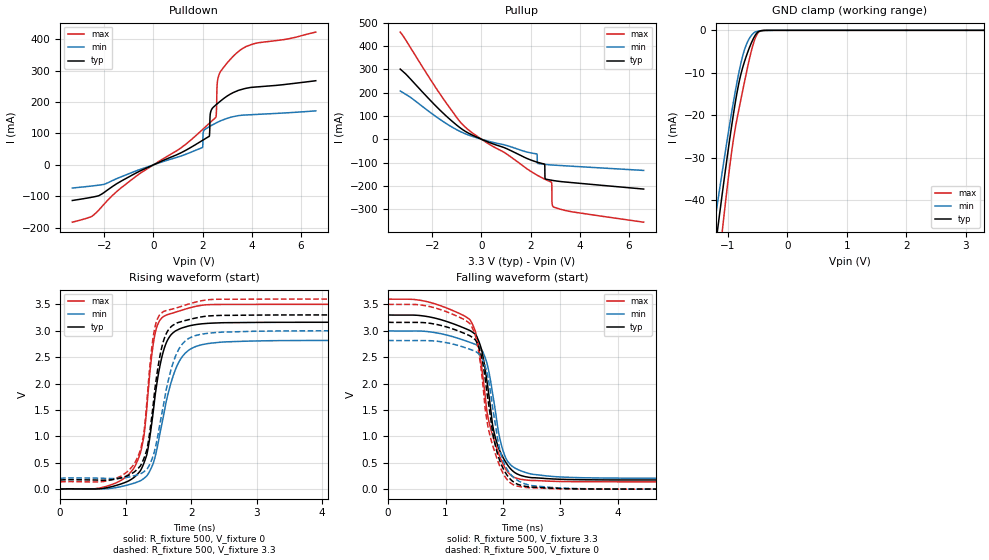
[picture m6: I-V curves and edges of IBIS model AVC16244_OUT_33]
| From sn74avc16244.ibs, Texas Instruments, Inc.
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[Model]   AVC16244_OUT_33
Model_type  3-state
Enable   Active-Low
Vref =   0
Rref =   500
Cref =   50p
Vmeas =   1.5
| variable   typ   min   max
C_comp   4.23pF   3.26pF   5.24pF
| C_pullup   8.74pF   0.03pF   34.91pF
| C_pulldown   15.41pF   1.21pF   46.75pF
| C_tri-state   4.23pF   3.26pF   5.24pF
[Temperature Range]   40   100   -40
| Ambient temperature   25   85   -40
[Voltage range]   3.3   3   3.6
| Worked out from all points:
|   slope of the pulldown table from 0 to 0.495 V, typ, clamps not added: 28.5 ohm
|   slope of the pullup table from 0 to 0.495 V, typ, clamps not added: 23.7 ohm
|   GND clamp passes 1 mA (typ) near -0.53 V on its own axis
|   rising waveform, R_fixture 500, V_fixture 0: 20-80 % time 241ps typ, 318ps min, 200ps max; typ from 0 V to 3.16 V
|   falling waveform, R_fixture 500, V_fixture 3.3: 20-80 % time 299ps typ, 286ps min, 336ps max; typ from 3.3 V to 0.173 V
|   rising waveform, R_fixture 500, V_fixture 3.3: 20-80 % time 217ps typ, 289ps min, 182ps max; typ from 0.173 V to 3.3 V
|   falling waveform, R_fixture 500, V_fixture 0: 20-80 % time 292ps typ, 284ps min, 316ps max; typ from 3.16 V to 0 V
[GND Clamp]
| AVC16244_OUT_33
|   Voltage   I(typ)   I(min)   I(max)
-3.3V     -301.3mA   -262.3mA   -362.9mA
-1.23V    -53.11mA   -45.98mA   -64.91mA
-1.175V   -47.08mA   -40.74mA   -57.65mA
-1.15V    -44.37mA   -38.39mA   -54.38mA
-1.08V    -36.9mA    -31.89mA   -45.41mA
-935mV    -22.33mA   -19.15mA   -28.4mA
-815mV    -12.4mA    -9.921mA   -18.58mA
-690mV    -6.054mA   -3.375mA   -10.05mA
-545mV    -1.258mA   -418.4uA   -2.023mA
-485mV    -307.6uA   -164.9uA   -439.4uA
-370mV    -14.24uA   -20.26uA   -8.565uA
3.3V      1.015nA    11.4nA     48.3pA
[Pulldown]
| AVC16244_OUT_33
|   Voltage   I(typ)   I(min)   I(max)
-3.3V     -113.7mA   -73.92mA   -182.8mA
-2.49V    -103.1mA   -67.29mA   -163.5mA
1.99V     77.64mA    55mA       111.9mA
2.035V    79.8mA     106.5mA    115.2mA
2.26V     90.24mA    120.9mA    131.5mA
2.32V     166.2mA    123.7mA    135.8mA
2.53V     190.2mA    132.7mA    150.5mA
2.555V    191.9mA    133.7mA    161.2mA
2.59V     194.3mA    135mA      255.5mA
2.66V     198.9mA    137.7mA    285.6mA
3.485V    238mA      157mA      362.9mA
6.6V      267.9mA    171.9mA    422.9mA
[Pullup]
| AVC16244_OUT_33
|   Voltage   I(typ)   I(min)   I(max)
-3.3V     300.9mA    206.8mA    459.7mA
-730mV    38.94mA    26.73mA    59.5mA
2.255V    -98.11mA   -63.13mA   -153.5mA
2.28V     -98.9mA    -103mA     -155mA
2.565V    -106.8mA   -107.8mA   -170.9mA
2.595V    -168.1mA   -108.1mA   -172.4mA
2.85V     -176mA     -110.5mA   -184.7mA
2.865V    -176.3mA   -110.6mA   -197.1mA
2.87V     -176.4mA   -110.7mA   -265.4mA
2.875V    -176.5mA   -110.7mA   -275.7mA
2.925V    -177.3mA   -111.1mA   -290.3mA
6.6V      -213.9mA   -134mA     -356.1mA
[Ramp]
| AVC16244_OUT_33
| variable   typ   min   max
dV/dt_r   1.90/2.43E-10   1.69/3.24E-10   2.10/2.01E-10
dV/dt_f   1.88/3.02E-10   1.68/2.94E-10   2.08/3.41E-10
R_load = 500
[Rising Waveform]
| AVC16244_OUT_33
R_fixture =   500
C_fixture =   0
L_fixture =   0
V_fixture =   0
V_fixture_min = 0
V_fixture_max = 0
|   Time   V(typ)   V(min)   V(max)
0s        34.29nV    120.2nV    1.957nV
1.03ns    146.5mV    78.97mV    260.1mV
1.225ns   347.7mV    158.5mV    680.3mV
1.325ns   659.2mV    253.7mV    1.561V
1.39ns    1.164V     395.7mV    2.438V
1.45ns    1.765V     611.3mV    2.945V
1.625ns   2.783V     1.686V     3.299V
1.845ns   3.046V     2.474V     3.384V
2.205ns   3.135V     2.746V     3.489V
29.99ns   3.161V     2.817V     3.501V
[Falling Waveform]
| AVC16244_OUT_33
R_fixture =   500
C_fixture =   0
L_fixture =   0
V_fixture =   3.3
V_fixture_min = 3
V_fixture_max = 3.6
|   Time   V(typ)   V(min)   V(max)
0s        3.3V       3V         3.6V
710ps     3.264V     2.982V     3.543V
1.425ns   3.004V     2.78V      3.207V
1.555ns   2.862V     2.719V     2.819V
1.7ns     2.201V     2.458V     1.667V
1.815ns   1.244V     1.84V      1.034V
1.895ns   871.9mV    1.275V     763.5mV
2.065ns   481.3mV    554.6mV    351.9mV
2.39ns    236mV      316.4mV    174.2mV
29.99ns   173.2mV    206mV      138.4mV
[Rising Waveform]
| AVC16244_OUT_33
R_fixture =   500
C_fixture =   0
L_fixture =   0
V_fixture =   3.3
V_fixture_min = 3
V_fixture_max = 3.6
|   Time   V(typ)   V(min)   V(max)
0s        173.2mV    206mV      138.4mV
1.035ns   257.5mV    226.5mV    341.8mV
1.225ns   439.6mV    290.2mV    737.8mV
1.28ns    584.9mV    331.4mV    1.081V
1.325ns   749mV      376.7mV    1.664V
1.445ns   1.873V     740.8mV    3.049V
1.62ns    2.943V     1.883V     3.382V
1.85ns    3.172V     2.724V     3.462V
2.265ns   3.28V      2.953V     3.588V
29.99ns   3.3V       3V         3.6V
[Falling Waveform]
| AVC16244_OUT_33
R_fixture =   500
C_fixture =   0
L_fixture =   0
V_fixture =   0
V_fixture_min = 0
V_fixture_max = 0
|   Time   V(typ)   V(min)   V(max)
0s        3.161V     2.817V     3.501V
745ps     3.139V     2.811V     3.453V
1.425ns   2.904V     2.649V     3.134V
1.56ns    2.74V      2.579V     2.702V
1.69ns    2.09V      2.328V     1.529V
1.76ns    1.536V     1.99V      1.074V
1.885ns   746mV      1.102V     611.1mV
2.06ns    282.3mV    397.6mV    197.6mV
2.38ns    55.35mV    101mV      34.19mV
29.99ns   24.63nV    158.8nV    -1.544nV
